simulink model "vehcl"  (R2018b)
settings: Solver=VariableStepAuto  StartTime=0.0  StopTime=200  RelTol=1e-3
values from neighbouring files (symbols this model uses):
  z0 = [0;20]    [initialization.m]

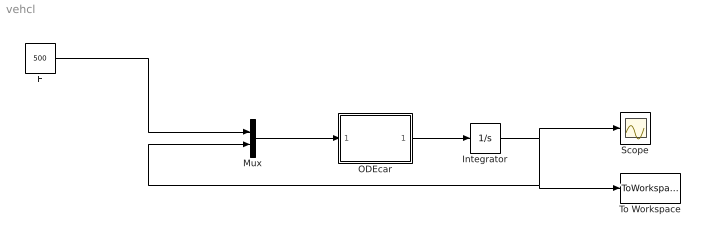
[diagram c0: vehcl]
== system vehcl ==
  F : Constant  Value=500
  Integrator : Integrator  InitialCondition=z0
  Mux : Mux  Inputs=2
  ODEcar : MATLAB Function  TreatAsAtomicUnit=on
  Scope : Scope
  To Workspace : ToWorkspace  VariableName=z  SampleTime=-1
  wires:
  F/1 -> Mux/1
  Mux/1 -> ODEcar/1(u)
  ODEcar/1(y) -> Integrator/1
  Integrator/1 -> To Workspace/1, Mux/2, Scope/1

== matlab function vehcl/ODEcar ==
function y = ODEcar(u)
% Constant
m = 1000;  % mass  % mass
% Parameters
k = 50; % Gain (m/s % pedal)

F = u(1);
x = u(2);
v = u(3);

% ODE equation 
dxdt = v;
dvdt =  (F - k * v )/ m;

y = [dxdt; dvdt];
